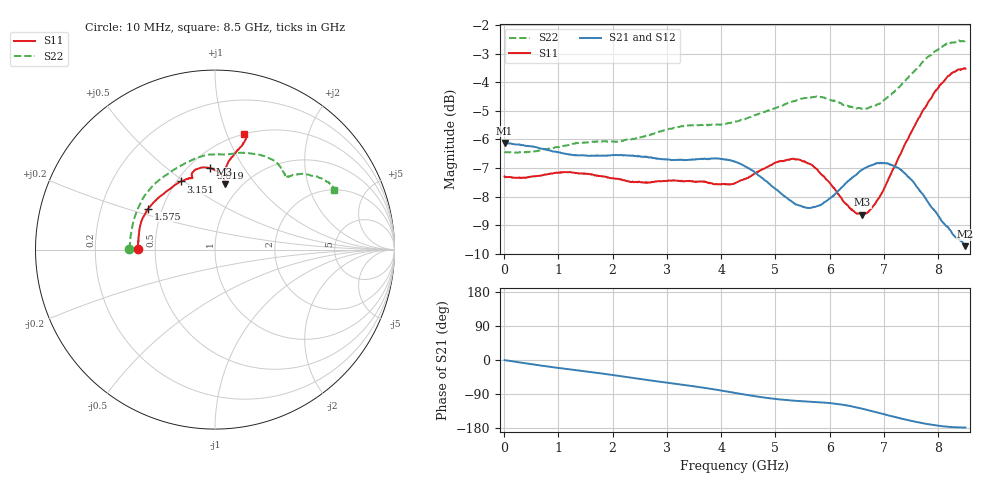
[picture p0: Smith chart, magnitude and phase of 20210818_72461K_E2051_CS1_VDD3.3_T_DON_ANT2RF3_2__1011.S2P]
!Agilent Technologies,E5071C,MY46417908,A.11.23
!Date: Wed Aug 18 14:30:58 2021
!Data & Calibration Information:
!Freq	S11:SOLT2(ON)	S21:SOLT2(ON)	S12:SOLT2(ON)	S22:SOLT2(ON)
!PortZ  Port1:50+j0  Port2:50+j0
!Above PortZ is port z conversion or system Z0 setting when saving the data.
!When reading, reference impedance value at option line is always used.
# Hz S dB R 50
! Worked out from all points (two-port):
!   1601 points, 10 MHz to 8.5 GHz, reference 50 ohm
!   highest |S21| = -6.12 dB at 10 MHz (marker M1); lowest = -9.7 dB at 8.5 GHz (marker M2)
!   |S21| within 3 dB of the highest: start of sweep to 8.197 GHz
!   lowest |S11| = -8.6 dB at 6.6 GHz (marker M3), VSWR 2.18, Z = 41.9 + j35.5 ohm
!   |S11| at or under -10 dB: nowhere
!   |S22| runs from -6.5 to -2.5 dB; largest |S21 - S12| = 0.0028
!   S11 on the Smith chart (normalised r, x): 10 MHz: 0.40, +0.00; 1.575 GHz: 0.42, +0.24; 3.151 GHz: 0.53, +0.49; 5.619 GHz: 0.63, +0.72; 8.5 GHz: 0.50, +1.15
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1e7  -7.30 179.7  -6.12 -0.4  -6.12 -0.3  -6.42 179.6
7.847125e8  -7.22 165.1  -6.36 -16.8  -6.36 -16.9  -6.33 158.9
1.426769e9  -7.19 151.7  -6.55 -28.8  -6.56 -28.7  -6.11 140.2
1.575344e9  -7.21 148.4  -6.57 -31.5  -6.58 -31.5  -6.10 135.8
2.238625e9  -7.44 134.5  -6.56 -44.5  -6.56 -44.5  -6.02 118.0
2.843538e9  -7.46 122.0  -6.67 -56.8  -6.67 -56.9  -5.74 104.0
3.1513e9  -7.44 116.6  -6.72 -62.7  -6.72 -62.7  -5.60 98.0
3.634169e9  -7.48 109.8  -6.69 -72.3  -6.68 -72.4  -5.50 89.5
4.255e9  -7.53 107.4  -6.78 -86.8  -6.77 -86.8  -5.38 81.3
4.663581e9  -7.14 107.2  -7.22 -96.4  -7.21 -96.4  -5.12 76.5
5.008488e9  -6.81 104.5  -7.74 -102.9  -7.75 -102.9  -4.90 70.8
5.618706e9  -6.84 93.2  -8.39 -109.8  -8.41 -109.8  -4.54 58.7
5.671769e9  -6.90 92.3  -8.38 -110.2  -8.41 -110.2  -4.53 57.7
6.08035e9  -7.69 84.2  -7.94 -114.8  -7.95 -115.0  -4.63 51.0
6.33505e9  -8.31 81.6  -7.46 -120.4  -7.46 -120.7  -4.83 47.6
6.600362e9  -8.63 81.8  -7.06 -128.6  -7.05 -128.7  -4.93 45.8
6.812612e9  -8.31 82.6  -6.88 -136.1  -6.88 -136.1  -4.85 45.2
7.088538e9  -7.36 82.9  -6.86 -146.4  -6.86 -146.4  -4.49 44.0
7.497119e9  -5.77 80.1  -7.40 -160.4  -7.40 -160.5  -3.74 40.4
7.842025e9  -4.62 76.2  -8.28 -170.0  -8.25 -170.2  -3.08 35.3
8.165706e9  -3.82 74.5  -9.06 -175.9  -9.02 -176.0  -2.66 30.4
8.5e9  -3.53 76.0  -9.73 -178.4  -9.66 -178.4  -2.61 26.8
